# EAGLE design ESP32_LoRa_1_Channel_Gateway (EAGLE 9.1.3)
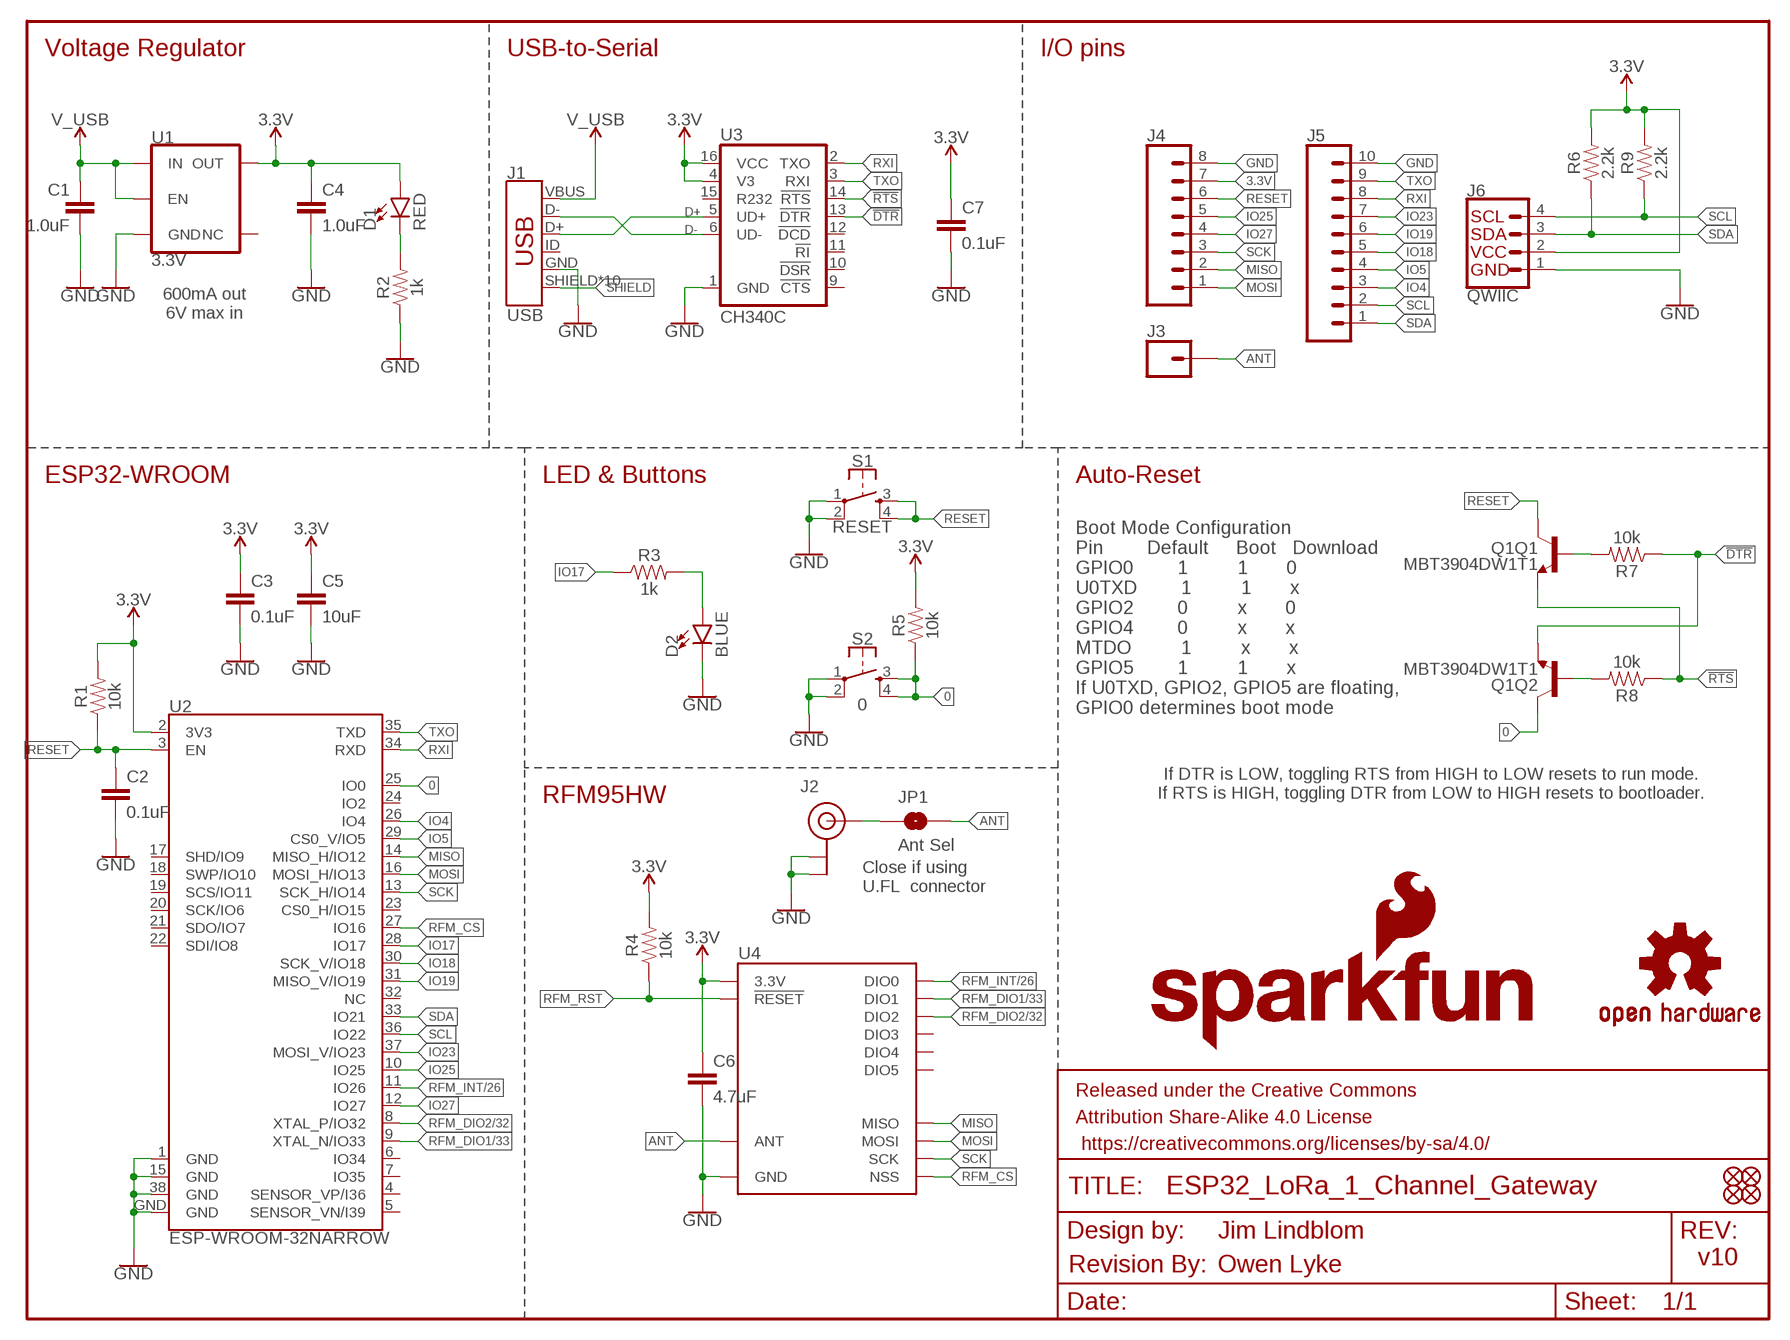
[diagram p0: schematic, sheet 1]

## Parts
C1  1.0uF  1.0UF-0603-16V-10%  [0603]
C2  0.1uF  0.1UF-0603-25V-(+80/-20%)  [0603]
C3  0.1uF  0.1UF-0603-25V-(+80/-20%)  [0603]
C4  1.0uF  1.0UF-0603-16V-10%  [0603]
C5  10uF  10UF-0603-6.3V-20%  [0603]
C6  4.7uF  4.7UF-0603-6.3V-(10%)  [0603]
C7  0.1uF  0.1UF-0603-25V-5%  [0603]
D1  RED  LED-RED0603  [LED-0603]
D2  BLUE  LED-BLUE0603  [LED-0603]
FD1  FIDUCIAL1X2  [FIDUCIAL-1X2]
FD2  FIDUCIAL1X2  [FIDUCIAL-1X2]
FD3  FIDUCIAL1X2  [FIDUCIAL-1X2]
FD4  FIDUCIAL1X2  [FIDUCIAL-1X2]
FRAME1  FRAME-LETTER  [CREATIVE_COMMONS]
J1  USB  USB_MICRO-B_HALF_PTH_MILL  [USB-MICROB-PTH-MILL]
J2  U.FL  [U.FL]
J3  CONN_01PTH_NO_SILK_YES_STOP  [1X01_NO_SILK]
J4  CONN_08NO_SILK_FEMALE_PTH  [1X08_NO_SILK]
J5  CONN_10NO_SILK_PTH_FEMALE  [1X10_NO_SILK]
J6  QWIIC  QWIIC_CONNECTORJS-1MM  [1X04_1MM_RA]
JP1  Ant Sel  JUMPER-SMT_2_NO_NO-SILK  [SMT-JUMPER_2_NO_NO-SILK]
LOGO1  REVISION  [REVISION]
LOGO2  SFE_LOGO_NAME_FLAME.1_INCH  [SFE_LOGO_NAME_FLAME_.1]
LOGO3  OSHW-LOGOS  [OSHW-LOGO-S]
Q1  MBT3904DW1T1  TRANS_NPN_DUAL-MBT3904DW1T1  [SC70-6]
R1  10k  10KOHM-0603-1/10W-1%  [0603]
R2  1k  1KOHM-0603-1/10W-1%  [0603]
R3  1k  1KOHM-0603-1/10W-1%  [0603]
R4  10k  10KOHM-0603-1/10W-1%  [0603]
R5  10k  10KOHM-0603-1/10W-1%  [0603]
R6  2.2k  2.2KOHM-0603-1/10W-1%  [0603]
R7  10k  10KOHM-0603-1/10W-1%  [0603]
R8  10k  10KOHM-0603-1/10W-1%  [0603]
R9  2.2k  2.2KOHM-0603-1/10W-1%  [0603]
S1  RESET  MOMENTARY-SWITCH-SPST-2-SMD-4.6X2.8MM  [TACTILE_SWITCH_SMD_4.6X2.8MM]
S2  0  MOMENTARY-SWITCH-SPST-2-SMD-4.6X2.8MM  [TACTILE_SWITCH_SMD_4.6X2.8MM]
U1  3.3V  V_REG_AP2112K-3.3V  [SOT23-5]
U2  ESP-WROOM-32NARROW  [ESP-WROOM-32-NARROW]
U3  CH340C  [SO016]
U4  RFM95W  [RFM95/96/97/98W]

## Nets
0: Q1.6(Q2:C) R5.1 S2.3 S2.4 U2.25(IO0)
3.3V: C3.1 C4.1 C5.1 C6.1 C7.1 D1.A J4.7 J6.2 R1.2 R4.2 R5.2 R6.2 R9.2 U1.5(OUT) U2.2(3V3) U3.4(V3) U3.16(VCC) U4.3.3V
!DTR: Q1.1(Q2:E) R7.1 U3.13(!DTR)
!RTS: Q1.4(Q1:E) R8.1 U3.14(!RTS)
ANT: J3.1 JP1.2 U4.ANT
D+: J1.D+ U3.5(UD+)
D-: J1.D- U3.6(UD-)
GND: C1.2 C2.2 C3.2 C4.2 C5.2 C6.2 C7.2 D2.C J1.GND J2.1(GND) J2.2(GND) J4.8 J5.10 J6.1 R2.1 S1.1 S1.2 S2.1 S2.2 U1.2(GND) U2.1(GND) U2.15(GND) U2.38(GND) U2.GND U3.1(GND) U4.GND@1(GND) U4.GND@2(GND) U4.GND@3(GND)
IO4: J5.3 U2.26(IO4)
IO5: J5.4 U2.29(CS0_V/IO5)
IO17: R3.1 U2.28(IO17)
IO18: J5.5 U2.30(SCK_V/IO18)
IO19: J5.6 U2.31(MISO_V/IO19)
IO23: J5.7 U2.37(MOSI_V/IO23)
IO25: J4.5 U2.10(IO25)
IO27: J4.4 U2.12(IO27)
MISO: J4.2 U2.14(MISO_H/IO12) U4.MISO
MOSI: J4.1 U2.16(MOSI_H/IO13) U4.MOSI
N$1: D1.C R2.2
N$2: D2.A R3.2
N$3: J2.FEED(SIGNAL) JP1.1
N$10: Q1.5(Q1:B) R7.2
N$12: Q1.2(Q2:B) R8.2
RESET: C2.1 J4.6 Q1.3(Q1:C) R1.1 S1.3 S1.4 U2.3(EN)
RFM_CS: U2.27(IO16) U4.NSS
RFM_DIO1/33: U2.9(XTAL_N/IO33) U4.DIO1
RFM_DIO2/32: U2.8(XTAL_P/IO32) U4.DIO2
RFM_INT/26: U2.11(IO26) U4.DIO0
RFM_RST: R4.1 U4.!RESET
RXI: J5.8 U2.34(RXD) U3.2(TXO)
SCK: J4.3 U2.13(SCK_H/IO14) U4.SCK
SCL: J5.2 J6.4 R9.1 U2.36(IO22)
SDA: J5.1 J6.3 R6.1 U2.33(IO21)
SHIELD: J1.SHIELD J1.SHIELD2(SHIELD) J1.SHIELD3(SHIELD) J1.SHIELD4(SHIELD) J1.SHIELD5(SHIELD) J1.SHIELD6(SHIELD) J1.SHIELD7(SHIELD) J1.SHIELD8(SHIELD) J1.SHIELD9(SHIELD) J1.SHIELD10(SHIELD)
TXO: J5.9 U2.35(TXD) U3.3(RXI)
V_USB: C1.1 J1.VBUS U1.1(IN) U1.3(EN)
Unconnected: J1.ID U1.4(NC) U2.4(SENSOR_VP/I36) U2.5(SENSOR_VN/I39) U2.6(IO34) U2.7(IO35) U2.17(SHD/IO9) U2.18(SWP/IO10) U2.19(SCS/IO11) U2.20(SCK/IO6) U2.21(SDO/IO7) U2.22(SDI/IO8) U2.23(CS0_H/IO15) U2.24(IO2) U2.32(NC) U3.9(!CTS) U3.10(!DSR) U3.11(!RI) U3.12(!DCD) U3.15(R232) U4.DIO3 U4.DIO4 U4.DIO5

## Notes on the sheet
- Voltage Regulator | USB-to-Serial | I/O pins
- 600mA out
  6V max in
- ESP32-WROOM | LED & Buttons | Auto-Reset
- Boot Mode Configuration
  Pin        Default     Boot   Download
  GPIO0        1         1       0
  U0TXD        1         1       x
  GPIO2        0         x       0
  GPIO4        0         x       x
  MTDO         1         x       x
  GPIO5        1         1       x
  If U0TXD, GPIO2, GPIO5 are floating, 
  GPIO0 determines boot mode
- If DTR is LOW, toggling RTS from HIGH to LOW resets to run mode.
  If RTS is HIGH, toggling DTR from LOW to HIGH resets to bootloader.
- RFM95HW
- Close if using
  U.FL  connector
- Jim Lindblom
- v10
- Owen Lyke

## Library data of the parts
C1 C4 = SparkFun-Capacitors:1.0UF: 1µF ceramic capacitors; PROD_ID: CAP-00868
C2 C3 = SparkFun-Capacitors:0.1UF: 0.1µF ceramic capacitors; PROD_ID: CAP-00810
C5 = SparkFun-Capacitors:10UF: 10.0µF ceramic capacitors; PROD_ID: CAP-11015
C6 = SparkFun-Capacitors:4.7UF: 4.7µF ceramic capacitors; PROD_ID: CAP-08280
C7 = SparkFun-Capacitors:0.1UF: 0.1µF ceramic capacitors; PROD_ID: CAP-08604
D1 = SparkFun-LED:LED-RED: Red SMD LED; PROD_ID: DIO-00819
D2 = SparkFun-LED:LED-BLUE: Blue SMD LED; PROD_ID: DIO-08575
FD1-FD4 = SparkFun-Aesthetics:FIDUCIAL: Fiducial Alignment Points
FRAME1 = SparkFun-Aesthetics:FRAME-LETTER: Schematic Frame - Letter
J1 = SparkFun-Connectors:USB_MICRO-B: USB Type Micro-B Connector Male/female and PTH/SMT variants SparkFun Products: SparkFun microB USB Breakout SparkFun USB microB Plug Breakout SparkFun ESP8266 Thing; PROD_ID: CONN-13711
J2 = SparkFun-Connectors:U.FL: SMD Antenna Connector - U.FL 2mm height, 3.0mm x 3.0mm receptacle size. SparkFun Products: SparkFun WiFi Shield - ESP8266 SparkFun ESP8266 Thing SparkFun MiniGen - Pro Mini Signal Generator Shield; PROD_ID: CONN-09193; SF_ID: WRL-09144
J3 = SparkFun-Connectors:CONN_01: Single connection point. Often used as Generic Header-pin footprint for 0.1 inch spaced/style header connections
J4 = SparkFun-Connectors:CONN_08: Multi connection point. Often used as Generic Header-pin footprint for 0.1 inch spaced/style header connections On any of the 0.1 inch spaced packages, you can populate with these: Break Away Headers - Straight (PRT-00116) Break Away Male Headers - Right Angle (PRT-00553) Female Headers (PRT-00115)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; PROD_ID: CONN-08438
J5 = SparkFun-Connectors:CONN_10: Multi connection point. Often used as Generic Header-pin footprint for 0.1 inch spaced/style header connections On any of the 0.1 inch spaced packages, you can populate with these: Break Away Headers - Straight (PRT-00116) Break Away Male Headers - Right Angle (PRT-00553) Female Headers (PRT-00115)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; PROD_ID: CONN-11563
J6 = SparkFun-Connectors:QWIIC_CONNECTOR: SparkFun I2C Standard Qwiic Connector An SMD 1mm pitch JST connector makes it easy and quick (get it? Qwiic?) to connect I2C devices to each other. The Qwiic system enables fast and solderless connection between popular platforms and various sensors and actuators. We carry 200mm, 100mm, 50mm, and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; PROD_ID: CONN-13694
JP1 = SparkFun-Jumpers:JUMPER-SMT_2_NO: Normally open jumper
LOGO1 = SparkFun-Aesthetics:REVISION: "Revision By" Text
LOGO2 = SparkFun-Aesthetics:SFE_LOGO_NAME_FLAME: SparkFun Font Logo w/ Flame
LOGO3 = SparkFun-Aesthetics:OSHW-LOGO: Open-Source Hardware (OSHW) Logo
Q1 = SparkFun-DiscreteSemi:TRANS_NPN_DUAL: Dual NPN Transistors in Single Package The MBT3904W1 puts two general purpose 3904 NPN transistors in a single package. Datasheet SparkFun Products: SparkFun ESP32 Thing; PROD_ID: TRANS-13337
R1 R4 R5 R7 R8 = SparkFun-Resistors:10KOHM: 10kΩ resistor; PROD_ID: RES-00824
R2 R3 = SparkFun-Resistors:1KOHM: 1kΩ resistor; PROD_ID: RES-07856
R6 R9 = SparkFun-Resistors:2.2KOHM: 2.2kΩ resistor; PROD_ID: RES-08272
S1 S2 = SparkFun-Switches:MOMENTARY-SWITCH-SPST-2: Momentary Switch (Pushbutton) - SPST - Two Circuits Normally-open (NO) SPST momentary switches (buttons, pushbuttons). Schematic symbol includes two switch circuits. Variants SMD-4.6MMX2.8MM - 4.60mm x 2.80mm Tactile Momentary Button Switch - Used on SparkFun SAMD21 Mini Breakout SMD-5.2MM - Mini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; PROD_ID: SWCH-13065
U1 = SparkFun-IC-Power:V_REG_AP2112: AP2112 - 600mA CMOS LDO Regulator w/ Enable The AP2112 is CMOS process low dropout linear regulator with enable function, the regulator delivers a guaranteed 600mA (min.) continuous load current. Features Output Voltage Accuracy: ±1.5% Output Current: 600mA (Min.) Foldback Short Current Protection: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; PROD_ID: VREG-12457
U2 = SparkFun-RF:ESP-WROOM-32; PROD_ID: IC-13849
U3 = SparkFun-IC-Comms:CH340C; PROD_ID: IC-14038
U4 = SparkFun-RF:RFM95W: RFM95/96/97/98 The RFM95/96/97/98(W) transceivers feature the LoRaTM long range modem that provides ultra-long range spread spectrum communication and high interference immunity whilst minimising current consumption. These devices also support high performance (G)FSK modes for systems including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; PROD_ID: IC-13959

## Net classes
0 default: width 0.152 mm, drill 0.305 mm
1 power: width 0.178 mm

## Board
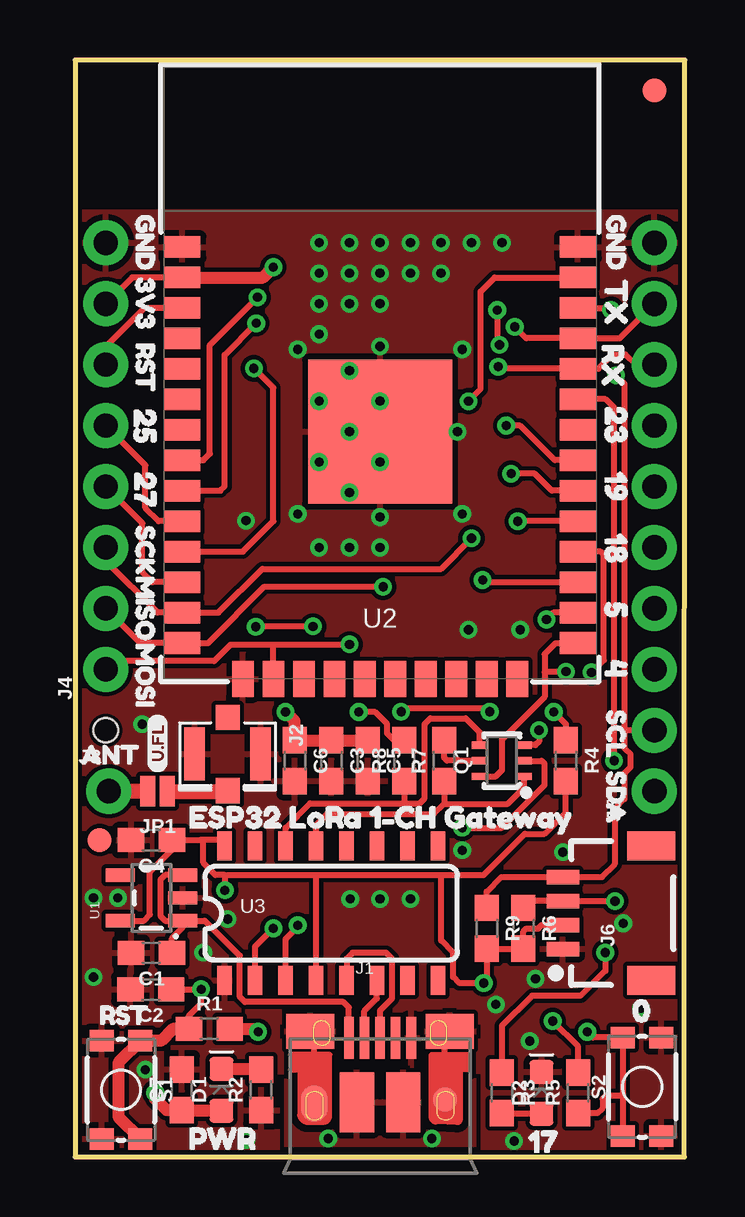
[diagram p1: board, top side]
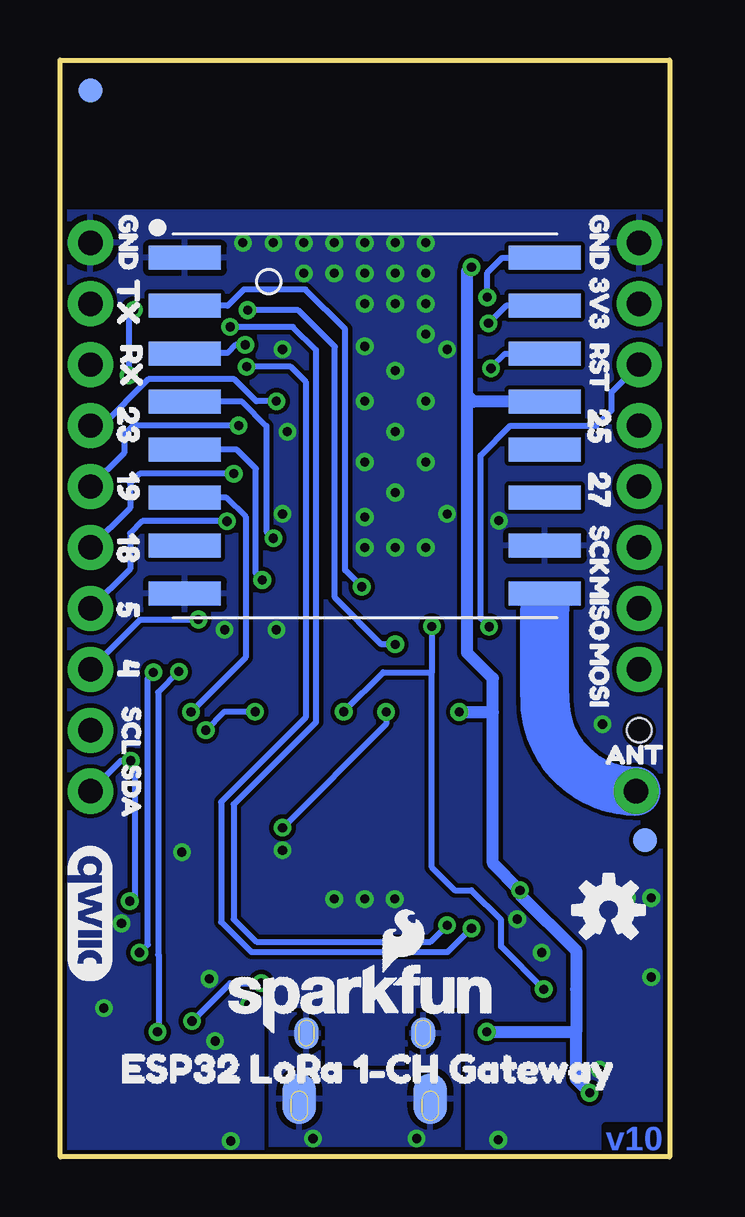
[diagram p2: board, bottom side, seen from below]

Size 25.4 x 45.72 mm. Coordinates in mm from the lower left corner, seen from the top.
Outline: 0,0 25.38,0 25.4,45.72 0,45.72 0,0
Copper layers (1*16): Top 0.035mm / dielectric 1.5mm / Bottom 0.035mm
Design rules "SparkFun-2-layer-TIGHT": minimum track width 7mil, minimum drill 15mil, track to track 7mil, track to pad 7mil, pad to pad 7mil, via to via 7mil, smd to smd 7mil, copper to edge 7mil, drill to drill 7mil, minimum pad ring 7mil, minimum via ring 7mil, stop-mask expansion 4mil, vias tented up to drill 25mil, thermal gap 10mil
Holes 1.02 mm at 1.27,17.78

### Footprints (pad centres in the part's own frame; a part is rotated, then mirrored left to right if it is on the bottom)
0603 = smd 1.1 x 1: 1 -0.85,0; 2 0.85,0
LED-0603 = smd 1 x 1: A -0.877,0; C 0.877,0
FIDUCIAL-1X2 = smd 1 x 1: 1 0,0
USB-MICROB-PTH-MILL = smd 0.4 x 1.75: D+ 0,0; D- -0.65,0; GND 1.3,0; ID 0.65,0; VBUS -1.3,0 | smd 2 x 1.46: SHIELD -2.9,0.275; SHIELD2 2.9,0.275 | smd 1.425 x 2.5: SHIELD3 -0.963,-2.675; SHIELD4 0.963,-2.675 | smd 1.4 x 2.1 bottom: SHIELD5 -2.731,-2.531; SHIELD7 2.729,-2.531 | smd 1 x 1: SHIELD6 2.7,-2.575 | smd 1.1 x 1.5: SHIELD8 -2.731,-2.731 | smd 1 x 1.3 bottom: SHIELD9 -2.43,0.195; SHIELD10 2.43,0.195
U.FL = smd 2.2 x 0.85: 1 0,1.375; 2 0,-1.375 | smd 1.05 x 1: FEED 1.525,0; NC -1.525,0
1X01_NO_SILK = drill 1.016 pad 1.88: 1 0,0
1X08_NO_SILK = drill 1.016 pad 1.88: 1 0,0; 2 2.54,0; 3 5.08,0; 4 7.62,0; 5 10.16,0; 6 12.7,0; 7 15.24,0; 8 17.78,0
1X10_NO_SILK = drill 1.016 pad 1.88: 1 0,0; 2 2.54,0; 3 5.08,0; 4 7.62,0; 5 10.16,0; 6 12.7,0; 7 15.24,0; 8 17.78,0; 9 20.32,0; 10 22.86,0
1X04_1MM_RA = smd 0.6 x 1.35: 1 -1.5,0; 2 -0.5,0; 3 0.5,0; 4 1.5,0 | smd 1.2 x 2: NC1 2.8,-3.675; NC2 -2.8,-3.675
SMT-JUMPER_2_NO_NO-SILK = smd 0.635 x 1.27: 1 -0.406,0; 2 0.406,0
SC70-6 = smd 0.3 x 0.66: 1 -0.65,-0.92; 2 0,-0.92; 3 0.65,-0.92; 4 0.65,0.92; 5 0,0.92; 6 -0.65,0.92
TACTILE_SWITCH_SMD_4.6X2.8MM = smd 0.9 x 1: 1 -2.05,-0.8; 2 2.05,-0.8; 3 2.05,0.8; 4 -2.05,0.8
SOT23-5 = smd 0.55 x 1.2: 1 -0.95,-1.3; 2 0,-1.3; 3 0.95,-1.3; 4 0.95,1.3; 5 -0.95,1.3
ESP-WROOM-32-NARROW = smd 0.9 x 1.5: 1 6.43,8.238; 2 5.16,8.238; 3 3.89,8.238; 4 2.62,8.238; 5 1.35,8.238; 6 0.08,8.238; 7 -1.19,8.238; 8 -2.46,8.238; 9 -3.73,8.238; 10 -5,8.238; 11 -6.27,8.238; 12 -7.54,8.238; 13 -8.81,8.238; 14 -10.08,8.238; 25 -10.08,-8.238; 26 -8.81,-8.238; 27 -7.54,-8.238; 28 -6.27,-8.238; 29 -5,-8.238; 30 -3.73,-8.238; 31 -2.46,-8.238; 32 -1.19,-8.238; 33 0.08,-8.238; 34 1.35,-8.238; 35 2.62,-8.238; 36 3.89,-8.238; 37 5.16,-8.238; 38 6.43,-8.238 | smd 1.5 x 0.9: 15 -11.57,5.715; 16 -11.57,4.445; 17 -11.57,3.175; 18 -11.57,1.905; 19 -11.57,0.635; 20 -11.57,-0.635; 21 -11.57,-1.905; 22 -11.57,-3.175; 23 -11.57,-4.445; 24 -11.57,-5.715 | smd 6 x 6: GND -1.27,0
SO016 = smd 0.6 x 1.2: 1 -4.445,-2.8; 2 -3.175,-2.8; 3 -1.905,-2.8; 4 -0.635,-2.8; 5 0.635,-2.8; 6 1.905,-2.8; 7 3.175,-2.8; 8 4.445,-2.8; 9 4.445,2.8; 10 3.175,2.8; 11 1.905,2.8; 12 0.635,2.8; 13 -0.635,2.8; 14 -1.905,2.8; 15 -3.175,2.8; 16 -4.445,2.8
RFM95/96/97/98W = smd 3 x 1: 3.3V 7.5,1; !RESET -7.5,-3; ANT 7.5,-7; DIO0 7.5,3; DIO1 7.5,5; DIO2 7.5,7; DIO3 7.5,-3; DIO4 7.5,-1; DIO5 -7.5,-5; GND@1 -7.5,7; GND@2 -7.5,-7; GND@3 7.5,-5; MISO -7.5,5; MOSI -7.5,3; NSS -7.5,-1; SCK -7.5,1

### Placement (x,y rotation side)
C1  3.17,8.51 180 top
C2  3.15,6.99 180 top
C3  10.67,16.51 270 top
C4  3.17,13.21 180 top
C5  12.19,16.51 270 top
C6  9.14,16.51 270 top
C7  4.45,2.79 90 top
D1  6.1,2.79 90 top
D2  19.43,2.67 90 top
FD1  24.13,44.45 0 bottom
FD2  1.02,13.21 0 top
FD3  24.13,44.45 0 top
FD4  1.02,13.21 0 bottom
FRAME1  not placed on the board
J1  12.7,4.95 0 top
J2  6.35,16.79 270 top
J3  1.4,15.24 0 top
J4  1.27,20.32 90 top
J5  24.13,15.24 90 top
J6  20.32,10.16 90 top
JP1  3.43,15.24 180 top
LOGO1  not placed on the board
LOGO2  18.8,5.08 0 bottom
LOGO3  2.54,10.29 0 bottom
Q1  17.78,16.51 90 top
R1  5.59,5.33 0 top
R2  7.75,2.79 90 top
R3  17.78,2.67 270 top
R4  20.45,16.51 270 top
R5  20.95,2.67 90 top
R6  18.67,9.53 270 top
R7  15.37,16.51 90 top
R8  13.72,16.51 90 top
R9  17.14,9.53 270 top
S1  1.91,2.79 270 top
S2  23.62,2.92 90 top
U1  3.17,10.79 90 top
U2  12.7,31.5 90 top
U3  10.67,10.16 0 top
U4  12.7,30.48 0 bottom
U$1  [GND0]  2.92,39.94 270 top
U$2  [3V31]  2.92,37.34 270 top
U$3  [RST2]  2.92,34.61 270 top
U$4  [2517]  2.92,32 270 top
U$5  [279]  2.92,29.34 270 top
U$6  [SCK3]  2.92,26.99 270 top
U$7  [MISO4]  2.92,24.89 270 top
U$8  [MOSI5]  2.92,22.1 270 top
U$9  [ANT6]  -0.48,16.76 0 top
U$10  [GND0]  22.54,39.94 270 top
U$11  [TX16]  22.54,37.34 270 top
U$12  [RX15]  22.42,34.67 270 top
U$13  [2314]  22.54,32.07 270 top
U$14  [1912]  22.54,29.34 270 top
U$15  [1811]  22.54,26.8 270 top
U$16  [513]  22.54,23.94 270 top
U$17  [410]  22.54,21.53 270 top
U$18  [SCL8]  22.54,19.3 270 top
U$19  [SDA7]  22.54,16.76 270 top
U$20  [RST2]  0.32,5.91 0 top
U$21  [020]  22.42,6.1 0 top
U$22  [PWR19]  3.94,0.76 0 top
U$23  [1722]  18.1,0.64 0 top
U$24  [U#FL0]  3.43,16 90 top
U$25  [ESP32_LORA_1#CH_GATEWAY21]  3.94,14.16 0 top
U$26  [GND0]  22.54,39.94 270 bottom
U$27  [TX16]  22.54,37.34 270 bottom
U$28  [RX15]  22.42,34.67 270 bottom
U$29  [2314]  22.54,32.07 270 bottom
U$30  [1912]  22.54,29.34 270 bottom
U$31  [1811]  22.54,26.8 270 bottom
U$32  [513]  22.54,23.94 270 bottom
U$33  [410]  22.54,21.53 270 bottom
U$34  [SCL8]  22.42,19.43 270 bottom
U$35  [SDA7]  22.42,17.02 270 bottom
U$36  [ANT6]  3.4,16.76 0 bottom
U$37  [GND0]  2.92,39.94 270 bottom
U$38  [3V31]  2.92,37.34 270 bottom
U$39  [RST2]  2.92,34.61 270 bottom
U$40  [2517]  2.92,32 270 bottom
U$41  [279]  2.92,29.34 270 bottom
U$42  [SCK3]  2.92,26.99 270 bottom
U$43  [MISO4]  2.92,24.89 270 bottom
U$44  [MOSI5]  2.92,22.1 270 bottom
U$45  [ESP32_LORA_1#CH_GATEWAY23]  23.88,3.68 0 bottom
U$46  [QWIIC_COPYRIGHT_SMALL]  24.13,10.16 270 bottom

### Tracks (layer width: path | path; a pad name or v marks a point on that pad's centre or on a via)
0  (via drill 0.38)
  Top 0.254: 22.82,2.54 S2.3 21.57,4.97 v21.34,5.21 | 22.82,2.54 S2.4 | R5.1 21.76,1.82 21.97,2.03 21.97,2.41 22.1,2.54 22.82,2.54 | U2.25 20.02,21.42 19.56,20.95 19.56,20.19 | 19.56,20.19 19.56,19.18 17.79,17.41 17.79,16.12 17.53,15.86 Q1.6 | 19.56,20.19 19.59,20.22 v20.45,20.22
  Bottom 0.254: v20.45,20.22 21.31,19.36 21.31,8.43 21.29,8.41 21.29,5.26 v21.34,5.21
3.3V  (via drill 0.38)
  Top 0.254: J4.7 2.37,36.66 U2.2 | R5.2 20.95,4.6 v19.9,5.66 | 6.22,11.74 5.84,11.74 5.33,12.25 5.33,13.21 | 6.22,11.74 10.03,11.74 | 10.03,11.74 15.24,11.74 | 6.22,11.74 6.22,11.12 v6.24,11.11 | U3.16 5.97,13.21 5.33,13.21 | 5.33,13.21 5.21,13.21 C4.1 4.03,12.79 3.11,11.87 3.11,10.1 2.86,9.85 U1.5 | U3.4 10.03,11.74 | 15.24,11.74 15.24,9.02 15.75,8.51 15.75,7.49 16,7.24 v17.02,7.24 17.14,7.37 R9.2 R6.2 18.67,9.39 18.8,9.52 19.3,9.52 19.43,9.66 J6.2 | 15.24,11.74 17.02,11.74 18.73,13.46 19.56,13.46 20.45,14.35 R4.2
  Top 0.508: v8.26,37.08 7.83,36.66 U2.2 | v8.76,18.54 9.14,18.16 C6.1 C3.1 C5.1 | R1.2 7.49,5.33 v7.62,5.21 | D1.A 4.47,1.92 C7.1 3.81,1.94 3.34,2.41 3.33,2.41 v3.33,2.67
  Bottom 0.254: v17.02,7.24 18.31,7.24 v19.9,5.66
  Bottom 0.508: v8.26,37.08 8.43,36.91 8.43,31.75 | 7.37,18.54 7.37,19.94 8.43,21.01 8.43,31.75 | v8.76,18.54 7.37,18.54 | 7.37,18.54 7.37,12.24 v6.24,11.11 6.24,10.95 3.9,8.61 3.9,6.99 3.9,5.21 | v7.62,5.21 3.9,5.21 | v3.33,2.67 3.9,3.23 3.9,5.21 | U4.3.3V 8.16,31.48 8.43,31.75
!DTR
  Top 0.254: Q1.1 18.7,15.4 18.02,14.72 15.37,14.72 | R7.1 15.37,14.72 | U3.13 10.03,13.84 10.49,14.3 14.95,14.3 15.37,14.72
!RTS
  Top 0.254: Q1.4 16.86,17.68 16.27,18.27 14.8,18.27 14.56,18.04 14.56,14.94 14.35,14.73 13.72,14.73 | R8.1 13.72,14.73 | U3.14 8.76,13.72 9.78,14.73 13.72,14.73
ANT
  Top 0.635: JP1.2 J3.1
  Bottom 1.016: 5.2,22.86 U4.ANT | 5.2,19.17 5.2,19.04
  Bottom 2.032: 5.2,19.04 arc-90 J3.1 | 5.2,19.17 5.2,22.86
D+
  Top 0.254: J1.D+ 12.7,6.1 13.21,6.6 13.21,8.26 12.95,8.51 11.56,8.51 11.3,8.26 U3.5
D-
  Top 0.254: J1.D- 12.05,6.08 12.57,6.6 U3.6
GND  (via drill 0.38)
  other vias: 12.7,33.78 12.7,26.67 17.78,38.1 9.27,26.8 9.27,33.66 16.51,38.1 16.13,33.66 2.92,3.63 18.94,4.83 23.57,6.2 7.11,26.52 15.93,30.23 16.13,26.8 7.14,0.71 19.18,7.42 10.16,25.4 0.76,10.79 1.78,10.79 15.24,38.1 13.97,38.1 12.7,38.1 11.43,38.1 10.16,38.1 15.24,36.83 13.97,36.83 12.7,36.83 11.43,36.83 10.16,36.83 12.7,35.56 11.43,35.56 10.16,35.56 10.16,34.29 0.76,7.49 18.54,21.97 16.38,21.97 11.43,25.4 12.7,25.4 2.79,18.03 11.46,10.74 12.7,10.74 13.97,10.74 17.53,6.35 16.13,12.78 20.32,12.7 18.29,0.66 22.83,9.73 5.33,8.51 11.43,32.77 12.7,31.5 10.16,31.5 11.43,30.23 12.7,28.96 10.16,28.96 11.43,27.69 6.35,9.91
  pour Top (isolate 0.152, rank 6): 0,0 0,39.37 25.4,39.37 25.4,0
  pour Bottom (isolate 0.152, rank 6): 25.4,0 25.4,39.37 0,39.37 0,0
IO4  (via drill 0.38)
  Top 0.254: U2.26 19.92,22.69 v19.63,22.4
  Bottom 0.254: J5.3 22.05,22.4 v19.63,22.4
IO5  (via drill 0.38)
  Top 0.254: U2.29 v18.44,26.5 v18.44,26.49
  Bottom 0.254: v18.44,26.49 21.97,26.49 22.48,25.98 22.48,24.51 J5.4
IO17  (via drill 0.38)
  Top 0.254: R3.1 17.78,5.46 19.04,6.72 21.06,6.72 22.09,7.75 v22.09,8.51 | U2.28 21.89,25.23 22.02,25.09 22.02,20.7 v21.51,20.19
  Bottom 0.254: v22.09,8.51 21.74,8.85 21.74,19.96 v21.51,20.19
IO18  (via drill 0.38)
  Top 0.254: U2.30 19.86,27.77 19.15,28.47 v18.16,28.47
  Bottom 0.254: v18.16,28.47 22.07,28.47 22.48,28.07 22.48,27.05 J5.5
IO19  (via drill 0.38)
  Top 0.254: U2.31 19.99,29.04 18.54,30.48 v17.96,30.48
  Bottom 0.254: v17.96,30.48 22.35,30.48 22.73,30.1 22.73,29.34 J5.6
IO23  (via drill 0.38)
  Top 0.254: v16.38,31.5 16.89,32 16.89,36.07 17.48,36.66 U2.37
  Bottom 0.254: v16.38,31.5 17.22,31.5 18.14,32.41 21.72,32.41 23.65,30.48 J5.7
IO25
  Top 0.254: U2.10 3.48,26.5 2.92,27.05 2.92,28.83 J4.5
IO27
  Top 0.254: U2.12 3.22,23.96 2.79,24.38 2.79,26.42 J4.4
MISO  (via drill 0.38)
  Top 0.254: J4.2 2.71,21.42 U2.14 5.54,21.42 7.88,23.76 v12.83,23.76
  Bottom 0.254: U4.MISO 18.41,35.48 17.74,36.16 15.18,36.16 13.52,34.5 13.52,24.45 v12.83,23.76
MOSI  (via drill 0.38)
  Top 0.254: 8.26,21.35 6.48,21.35 5.79,20.66 1.61,20.66 J4.1 | 8.26,21.35 11.42,21.35 v11.43,21.36 | U2.16 8.26,21.35 | v17.58,35.29 17.58,33.94 v17.68,33.85
  Bottom 0.254: v11.43,21.36 12.01,21.36 13.95,23.31 13.95,33.76 15.48,35.29 v17.58,35.29 | U4.MOSI 20.18,33.5 18.41,33.5 18.07,33.85 v17.68,33.85
N$1
  Top 0.508: R2.2 6.12,3.64 D1.C
N$2
  Top 0.254: D2.A 17.81,1.79 R3.2
N$3
  Top 0.635: JP1.1 6.33,15.24 arc90 J2.FEED
N$10
  Top 0.254: R7.2 15.37,16.64 15.49,16.52 15.99,16.52 16,16.51 Q1.5
N$12  (via drill 0.38)
  Top 0.254: Q1.2 19.43,16.51 19.56,16.38 19.56,15.49 17.78,13.72 v16.13,13.72 | R8.2 13.29,17.36 13,17.65 13,18.04 12.49,18.54 v11.81,18.54
  Bottom 0.254: v16.13,13.72 11.81,18.03 v11.81,18.54
RESET  (via drill 0.38)
  Top 0.254: U2.3 2.87,35.39 1.27,33.78 J4.6 | v9.91,22.11 7.53,22.11 v7.52,22.1 | v17.27,18.55 17.12,18.71 13.73,18.71 v13.58,18.55 | Q1.3 19.18,17.16 19.32,17.31 v19.32,17.78 | R1.1 4.74,5.88 5.25,6.39 v5.25,6.99 C2.1
  Top 0.508: S1.3 1.82,1.63 1.82,3.96 S1.4 3.57,4.84 4.06,5.33 R1.1
  Bottom 0.254: v9.91,22.11 9.91,20.19 | 9.91,20.19 9.91,12.06 8.95,11.11 8.26,11.11 7.02,9.88 7.02,8.76 v5.25,6.99 | J4.6 2.41,31.88 2.41,31.11 3.05,30.48 6.63,30.48 7.87,29.24 7.87,22.45 v7.52,22.1 | v13.58,18.55 11.94,20.19 9.91,20.19 | v19.32,17.78 18.55,18.55 v17.27,18.55
RFM_CS  (via drill 0.38)
  Top 0.254: U2.27 17.07,23.96 v16.98,24.05
  Bottom 0.254: U4.NSS 18.03,29.48 17.23,28.68 17.23,24.3 v16.98,24.05
RFM_DIO1/33  (via drill 0.38)
  Top 0.254: U2.9 6.05,27.77 6.22,27.94 6.22,33.43 v7.54,34.75
  Bottom 0.254: U4.DIO1 6.81,35.48 v7.54,34.75
RFM_DIO2/32  (via drill 0.38)
  Top 0.254: U2.8 5.33,29.04 5.61,29.31 5.61,33.84 v7.59,35.83
  Bottom 0.254: U4.DIO2 6.97,37.48 7.59,36.85 v7.59,35.83
RFM_INT/26  (via drill 0.38)
  Top 0.254: v7.44,32.87 8.26,32.05 8.26,26.5 6.99,25.23 U2.11
  Bottom 0.254: U4.DIO0 6.86,33.48 7.44,32.9 v7.44,32.87
RFM_RST  (via drill 0.38)
  Top 0.254: v19.94,18.54 20.45,18.03 R4.1
  Bottom 0.254: U4.!RESET 18.46,27.48 17.67,26.68 17.67,20.82 v19.94,18.54
RXI  (via drill 0.38)
  Top 0.254: v17.62,32.93 17.71,32.85 U2.34 21.8,32.85 22.4,33.45 22.92,33.45 23.35,33.02 J5.8 | v8.26,9.53 7.49,8.76 U3.2
  Bottom 0.254: v17.62,32.93 15.79,32.93 15.16,32.31 15.16,18.3 18.68,14.79 18.68,9.79 17.42,8.53 9.25,8.53 v8.26,9.53
SCK  (via drill 0.38)
  Top 0.254: v16.51,25.78 15.24,24.51 7.79,24.51 5.97,22.69 U2.13 3.43,22.69 1.27,24.84 J4.3
  Bottom 0.254: U4.SCK 17.82,31.48 16.8,30.47 16.8,26.07 v16.51,25.78
SCL  (via drill 0.38)
  Top 0.254: U2.36 22.24,35.39 v22.32,35.31 | v22.54,32.57 22.89,32.22 22.89,17.78 | 22.89,17.78 22.89,17.03 23.13,16.79 23.13,16.23 22.89,15.99 22.89,14.91 22.48,14.5 22.48,12.19 21.95,11.66 J6.4 17.76,11.66 17.14,11.05 R9.1 | J5.2 22.89,17.78
  Bottom 0.254: v22.32,35.31 22.54,35.09 v22.54,32.57
SDA  (via drill 0.38)
  Top 0.254: v22.49,10.66 J6.3 18.95,10.66 R6.1 | U2.33 22.1,31.58 22.45,31.22 v22.45,16.51
  Bottom 0.254: v22.49,10.66 22.29,10.86 22.29,16.34 v22.45,16.51 22.86,16.51 J5.1
SHIELD  (via drill 0.38)
  Top 0.254: J1.SHIELD6 15.4,5.03 J1.SHIELD2 | J1.SHIELD8 9.97,5.06 J1.SHIELD
  other vias: 10.54,0.76 14.86,0.76
  pour Top (isolate 0.305): 8.76,0 8.76,5.97 10.79,5.97 10.79,3.56 14.61,3.56 14.61,5.97 16.64,5.97 16.64,0.13 16.51,0
  pour Bottom (isolate 0.305): 16.64,0 16.64,5.97 14.61,5.97 14.61,3.56 10.79,3.56 10.79,5.97 8.76,5.97 8.76,0
TXO  (via drill 0.38)
  Top 0.254: v18.31,34.59 18.79,34.12 U2.35 22.69,34.12 J5.9 | U3.3 8.76,9.08 9.27,9.59 v9.27,9.65
  Bottom 0.254: v18.31,34.59 15.7,34.59 14.73,33.63 14.73,18.12 18.16,14.7 18.16,9.91 17.22,8.97 9.96,8.97 v9.27,9.65
V_USB
  Top 0.254: J1.VBUS 11.4,6.22 11.17,6.46 7.07,6.46 6.86,6.66 6.86,8.38 5.39,9.85 U1.1 | C1.1 4.03,9.11 4.47,9.55 U1.1 | U1.3 3.74,11.74 3.54,11.54 3.54,10.05 3.74,9.85 U1.1

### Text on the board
Bottom: v10
tDocu: Jim Lindblom | Owen Lyke

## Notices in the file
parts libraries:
SparkFun-Aesthetics: Licensing: Creative Commons ShareAlike 4.0 International - https://creativecommons.org/licenses/by-sa/4.0
SparkFun-Aesthetics: Released under the Creative Commons Attribution Share-Alike 4.0 License
SparkFun-Aesthetics: https://creativecommons.org/licenses/by-sa/4.0
